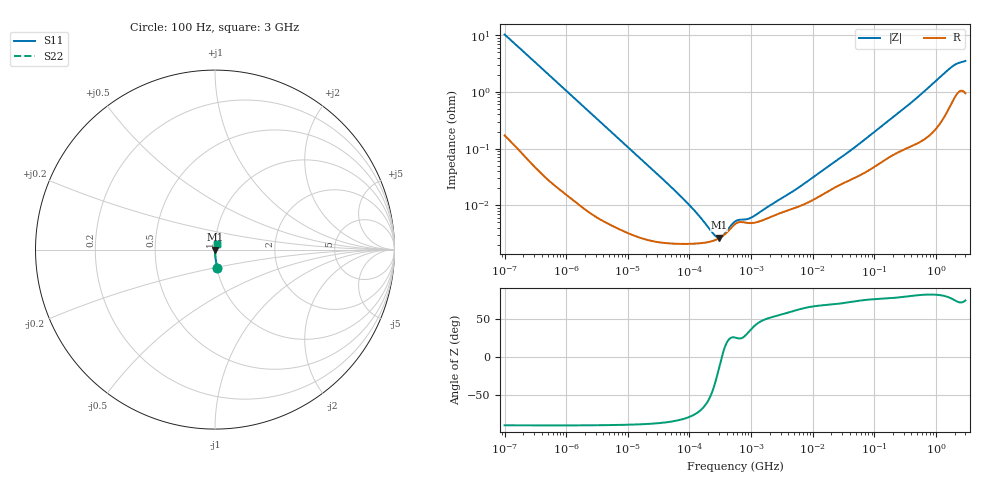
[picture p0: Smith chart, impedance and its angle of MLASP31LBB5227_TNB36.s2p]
! MLASP31LBB5227_TNB36  S-PARAMETER MODEL  ( Standard Model )
! Model Generated by TAIYO YUDEN Corporation (http://www.ty-top.com)
! Version 1.0
! TAIYO YUDEN Control No. 240524
! Copyright(c) 2024 TAIYO YUDEN CO.,LTD. All Rights Reserved.
! Product Description (link to TY-COMPAS)
! https://ds.yuden.co.jp/TYCOMPAS/or/detail?pn=MLASP31LBB5227MTNB36&u=M
! Products Name : Multilayer Ceramic Capacitors
! Characteristics :
!  Capacitance : 220 [uF] , Rated Voltage : 2.5 [V] , TCC : X5R
!  Case Size : 3.2 x 1.6 / 0.126 x 0.063 [mm/inch] , Thickness : 1.6 / 0.063 [mm/inch]
!  (Conditions: Temperature = 25 [degC] , DC Bias Voltage = 0 [V])
! External Node Assignments :
!  1  o---| |---o  2
! GND o---------o GND
! Frequency Range : 100Hz  -  3GHz  [ 401 STEP ]
# MHZ S RI R 50
! Freq[MHz].  S11 Real  S11 Imag  S21 Real  S21 Imag  S12 Real  S12 Imag  S22 Real  S22 Imag
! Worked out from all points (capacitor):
!   401 points, 100 Hz to 3 GHz, reference 50 ohm
!   read as one part in series: C = 154 uF near 109 Hz
!   lowest |Z| = 2.7 mohm at 299.8 kHz (marker M1)
!   series resonance near 333.6 kHz, so ESL is about 1.5 nH
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0.0001  0.0121 -0.1014  0.9879 0.1014  0.9879 0.1014  0.0121 -0.1014
0.000114  0.00957 -0.0895  0.9904 0.0895  0.9904 0.0895  0.00957 -0.0895
0.000175  0.00438 -0.0588  0.9956 0.0588  0.9956 0.0588  0.00438 -0.0588
0.000306  0.00163 -0.0339  0.9984 0.0339  0.9984 0.0339  0.00163 -0.0339
0.000664  0.000466 -0.0157  0.9995 0.0157  0.9995 0.0157  0.000466 -0.0157
0.001788  0.000128 -0.00589  0.9999 0.00589  0.9999 0.00589  0.000128 -0.00589
0.031977  2.24e-05 -0.000334  1 0.000334  1 0.000334  2.24e-05 -0.000334
0.09379  2.09e-05 -0.000106  1 0.000106  1 0.000106  2.09e-05 -0.000106
0.102221  2.1e-05 -9.59e-05  1 9.59e-05  1 9.59e-05  2.1e-05 -9.59e-05
0.111411  2.1e-05 -8.63e-05  1 8.63e-05  1 8.63e-05  2.1e-05 -8.63e-05
0.299821  2.61e-05 -6.87e-06  1 6.87e-06  1 6.87e-06  2.61e-05 -6.87e-06
0.547723  4.66e-05 2.26e-05  1 -2.26e-05  1 -2.26e-05  4.66e-05 2.26e-05
1.827928  5.89e-05 7.17e-05  0.9999 -7.17e-05  0.9999 -7.17e-05  5.89e-05 7.17e-05
2.079876  6.25e-05 8.01e-05  0.9999 -8.01e-05  0.9999 -8.01e-05  6.25e-05 8.01e-05
4.711951  8.71e-05 0.000152  0.9999 -0.000152  0.9999 -0.000152  8.71e-05 0.000152
9.794414  0.000122 0.000279  0.9999 -0.000279  0.9999 -0.000279  0.000122 0.000279
42.31884  0.000287 0.000905  0.9997 -0.000905  0.9997 -0.000905  0.000287 0.000905
175.1444  0.000714 0.00309  0.9993 -0.00309  0.9993 -0.00309  0.000714 0.00309
451.4794  0.00122 0.00718  0.9988 -0.00718  0.9988 -0.00718  0.00122 0.00718
1714.41  0.00635 0.0255  0.9937 -0.0255  0.9937 -0.0255  0.00635 0.0255
2219.584  0.0102 0.0297  0.9898 -0.0297  0.9898 -0.0297  0.0102 0.0297
3000  0.0105 0.0332  0.9895 -0.0332  0.9895 -0.0332  0.0105 0.0332
